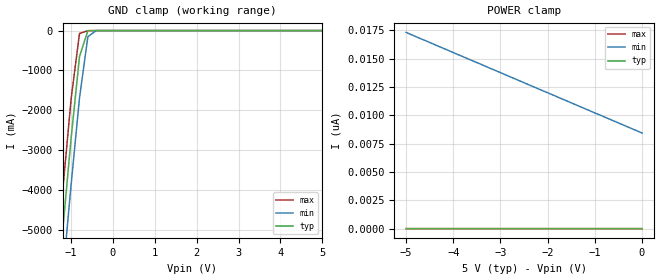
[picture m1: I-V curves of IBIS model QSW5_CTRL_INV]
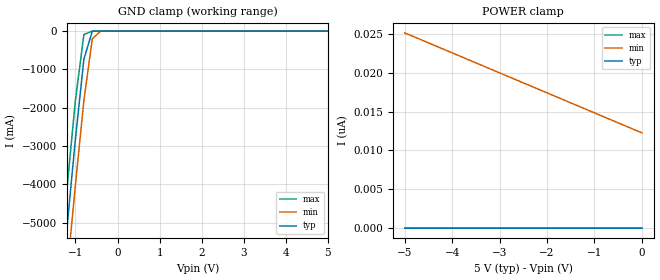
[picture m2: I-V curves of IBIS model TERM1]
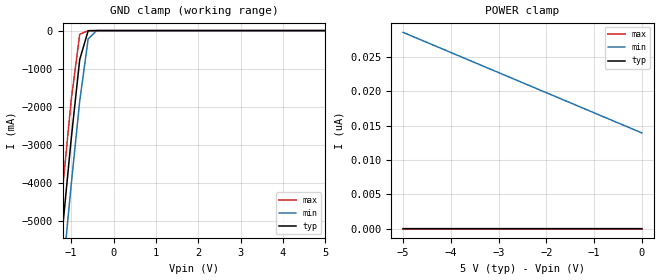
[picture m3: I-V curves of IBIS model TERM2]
| I/O Buffer Information Specification (IBIS) Version 3.2 (August 20, 1999)
| IBIS is a standard for electronic behavioral specifications of integrated
| circuit input/output analog characteristics.
[IBIS Ver]   3.2
[File Name]   qs3383.ibs
[File Rev]   1.0
[Date]   Wednesday, June 9, 2004
[Source]   Integrated Device Technology, Inc.
[Notes]   1.Temperatures: typ=25C, min=-40C, max=100C
[Disclaimer]
Integrated Device Technology, Inc. ("IDT") hereby grants the user of this
IBIS model ("User") a non-exclusive, nontransferable license to use this
IBIS model under the following terms: The User is granted this license only
to use the IBIS model for demonstration purposes only and is not granted
rights to sell, copy (except as needed to run the IBIS model), rent, lease
or sub-license (except for demonstration) the IBIS model in whole or in
part, or in modified form to anyone. The User may modify the IBIS model to
suit its specific applications, but  rights to derivative works and such
modifications shall belong to IDT.
THIS IBIS MODEL IS PROVIDED ON AN AS IS" BASIS AND IDT  MAKES ABSOLUTELY NO
WARRANTY WITH RESPECT TO THE INFORMATION CONTAINED HEREIN.  IDT DISCLAIMS
AND USER WAIVES ALL WARRANTIES, EXPRESS AND IMPLIED, INCLUDING WARRANTIES OF
MERCHANTABILITY AND FITNESS FOR A PARTICULAR PURPOSE.  THE ENTIRE RISK AS TO
QUALITY AND PERFORMANCE IS WITH THE USER  ACCORDINGLY, IN NO EVENT SHALL IDT
BE LIABLE FOR ANY DIRECT OR INDIRECT DAMAGES, WHETHER IN CONTRACT OR TORT,
INCLUDING ANY LOST PROFITS OR OTHER INCIDENTAL, CONSEQUENTIAL, EXEMPLARY, OR
PUNITIVE DAMAGES ARISING OUT OF THE USE OR APPLICATION OF THE  IBIS MODEL,
WHETHER OR NOT IDT HAD NOTICE OF SUCH DAMAGES.
IDT reserves the right to make changes without notice to any product herein
to improve reliability, function, or design. IDT does not convey any license
under patent rights or any other intellectual property rights, including those
of third parties. IDT is not obligated to provide maintenance or support for
the licensed IBIS model.
This model is for High-Speed CMOS 10-Bit Bus Exchange Switch
[Copyright]
Copyright 2002, Integrated Device Technology, Inc. All rights reserved.
|   Component qs3383
[Component]   qs3383
[Manufacturer]   Integrated Device Technology
[Package]
|Following package parameters are for TSSOP 24 lead package
| variable   typ   min   max
R_pkg   2.500m   2.44m   3.00m
L_pkg   1.00nH   0.91nH   1.74nH
C_pkg   0.17pF   0.16pF   0.27pF
[Pin]  signal_name   model_name   R_pin   L_pin   C_pin
1   _BEB_   QSW5_CTRL
2   C0   TERM2
3   A0   TERM1
4   B0   TERM1
5   D0   TERM2
6   C1   TERM2
7   A1   TERM1
8   B1   TERM1
9   D1   TERM2
10   C2   TERM2
11   A2   TERM1
12   GND   GND
13   BX   QSW5_CTRL
14   B2   TERM1
15   D2   TERM2
16   C3   TERM2
17   A3   TERM1
18   B3   TERM1
19   D3   TERM2
20   C4   TERM2
21   A4   TERM1
22   B4   TERM1
23   D4   TERM2
24   VCC   POWER
[Series Pin Mapping]   pin_2   model_name   function_table_group
3   2   QSW5_SW   A
7   6   QSW5_SW   A
11   10   QSW5_SW   A
17   16   QSW5_SW   A
21   20   QSW5_SW   A
4   5   QSW5_SW   A
8   9   QSW5_SW   A
14   15   QSW5_SW   A
18   19   QSW5_SW   A
22   23   QSW5_SW   A
3   5   QSW5_SW   B
7   9   QSW5_SW   B
11   15   QSW5_SW   B
17   19   QSW5_SW   B
21   23   QSW5_SW   B
4   2   QSW5_SW   B
8   6   QSW5_SW   B
14   10   QSW5_SW   B
18   16   QSW5_SW   B
22   20   QSW5_SW   B
|   Model QSW5_SW
[Model]   QSW5_SW
Model_type   Series_switch
C_comp   0.0pF   0.0pF   0.0pf
[Temperature Range]   25.00   100.00   -40.00
[Voltage Range]   5.00V   4.75V   5.25V
[On]
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[Off]
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| Models and submodels in the file (4): QSW5_CTRL_INV (Input), TERM1 (Input), TERM2 (Input), QSW5_SW (Series_switch)
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|   Model QSW5_CTRL_INV
[Model]   QSW5_CTRL_INV
Model_type   Input
Vinl =  0.80000V
Vinh =  2.00000V
C_comp   4.20000pF   4.20000pF   4.20000pF
[Temperature Range]   25.00000   100.00000   -40.00000
[Voltage Range]   5.00000V   4.75000V   5.25000V
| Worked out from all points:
|   GND clamp passes 1 mA (typ) near -0.48 V on its own axis
[GND_clamp]
| voltage   I(typ)   I(min)   I(max)
-5V       -51.74A    -52.8A     -50.85A
-1.4V     -7.368A    -8.538A    -6.375A
-1.2V     -4.993A    -6.169A    -3.993A
-1V       -2.692A    -3.858A    -1.708A
-800mV    -650.1mA   -1.689A    -70.61mA
-600mV    -2.541mA   -153.7mA   -3.31mA
-400mV    -3.914uA   -449.3uA   -30.03uA
5V        2.373pA    8.883nA    568.4fA
[POWER_clamp]
| voltage   I(typ)   I(min)   I(max)
-5V       3.268pA    17.31nA    739fA
-3.9V     3.055pA    15.35nA    710.5fA
-3.5V     2.998pA    14.65nA    682.1fA
0V        2.373pA    8.439nA    568.4fA
|   Model TERM1
[Model]   TERM1
Model_type   Input
Vinl =  0.80000V
Vinh =  2.00000V
C_comp   6.00000pF   6.00000pF   6.00000pF
[Temperature Range]   25.00000   100.00000   -40.00000
[Voltage Range]   5.00000V   4.75000V   5.25000V
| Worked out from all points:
|   GND clamp passes 1 mA (typ) near -0.46 V on its own axis
[GND_clamp]
| voltage   I(typ)   I(min)   I(max)
-5V       -51.86A    -52.95A    -50.94A
-1.4V     -7.483A    -8.681A    -6.464A
-1.2V     -5.106A    -6.309A    -4.081A
-1V       -2.799A    -3.993A    -1.789A
-800mV    -731.5mA   -1.811A    -88.62mA
-600mV    -3.518mA   -199.1mA   -2.949mA
-400mV    -5.218uA   -651.7uA   -27.72uA
5V        2.8pA      12.9nA     625.3fA
[POWER_clamp]
| voltage   I(typ)   I(min)   I(max)
-5V       4.036pA    25.11nA    824.2fA
-1V       3.041pA    14.83nA    667.9fA
-700mV    2.97pA     14.05nA    667.9fA
0V        2.8pA      12.26nA    639.5fA
|   Model TERM2
[Model]   TERM2
Model_type   Input
Vinl =  0.80000V
Vinh =  2.00000V
C_comp   6.00000pF   6.00000pF   6.00000pF
[Temperature Range]   25.00000   100.00000   -40.00000
[Voltage Range]   5.00000V   4.75000V   5.25000V
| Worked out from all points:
|   GND clamp passes 1 mA (typ) near -0.45 V on its own axis
[GND_clamp]
| voltage   I(typ)   I(min)   I(max)
-5V       -51.9A     -53A       -50.97A
-1.4V     -7.523A    -8.731A    -6.496A
-1.2V     -5.145A    -6.358A    -4.111A
-1V       -2.836A    -4.04A     -1.818A
-800mV    -760.5mA   -1.854A    -96.21mA
-600mV    -3.917mA   -216.8mA   -2.949mA
-400mV    -5.385uA   -741uA     -27.72uA
5V        2.927pA    14.67nA    625.3fA
[POWER_clamp]
| voltage   I(typ)   I(min)   I(max)
-5V       4.334pA    28.57nA    824.2fA
-4.1V     4.064pA    25.94nA    795.8fA
-3.7V     3.965pA    24.76nA    795.8fA
0V        2.927pA    13.94nA    639.5fA
